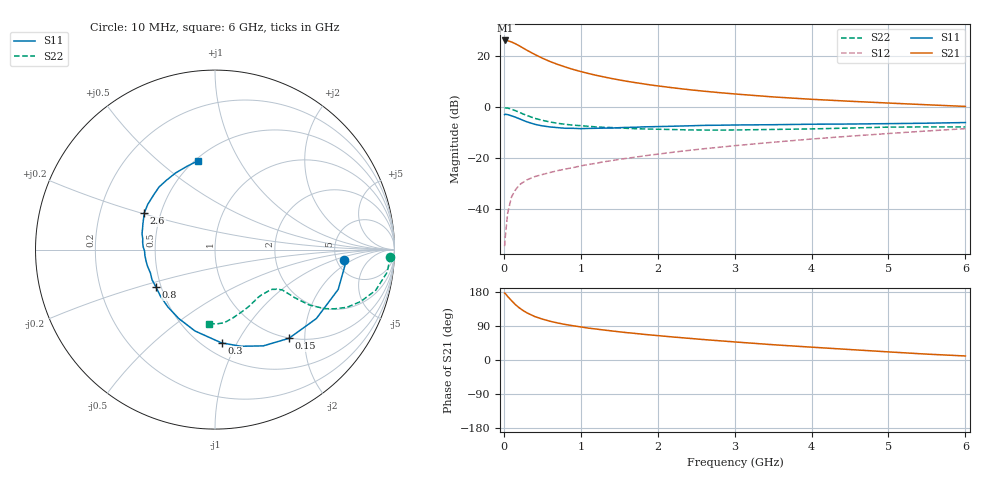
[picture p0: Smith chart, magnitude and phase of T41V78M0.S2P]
! Infineon Technologies  Discrete & RF Semiconductors
! BFR182T
! Si NPN RF Bipolar Junction Transistor in SC75
! VCE = 1.75 V  IC = 8 mA
! Common Emitter S-Parameters:  October  1999
# GHz  S  MA  R  50
!  f  S11  S21  S12  S22
! GHz  MAG  ANG  MAG  ANG  MAG  ANG  MAG  ANG
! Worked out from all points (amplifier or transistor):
!   36 points, 10 MHz to 6 GHz, reference 50 ohm
!   highest |S21| = 26.2 dB at 20 MHz (marker M1)
!   |S21| within 3 dB of that: start of sweep to 251.7 MHz
!   unconditionally stable (mu >= 1): 1.06 GHz to 3.891 GHz
!   at 250 MHz: K = 0.40, MSG = 26.3 dB, |S12| = -29.4 dB
!   at 1.4 GHz: K = 1.08, MAG = 14.4 dB, |S12| = -20.9 dB
!   at 6 GHz: K = 0.85, MSG = 4.4 dB, |S12| = -8.3 dB
!   lowest NFmin = 1.40 dB at 450 MHz
!   S11 on the Smith chart (normalised r, x): 10 MHz: 5.81, -1.47; 150 MHz: 0.99, -1.67; 300 MHz: 0.61, -0.87; 800 MHz: 0.47, -0.23; 2.6 GHz: 0.40, +0.21; 6 GHz: 0.52, +0.69
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0.01  0.722 -4.8  20.52 176.7  0.0019 84.7  0.9757 -2.3
0.02  0.7313 -6.0  20.52 175.3  0.003 95.7  0.9763 -3.0
0.05  0.7214 -17.9  20.27 167.7  0.0085 84.4  0.9674 -7.5
0.1  0.6832 -34.2  19.14 156.6  0.0176 75.7  0.9237 -14.2
0.15  0.6434 -50.2  17.7 146.2  0.0239 69.1  0.8622 -19.6
0.2  0.6 -63.4  16.15 137.7  0.0302 65.3  0.8029 -23.6
0.25  0.5575 -75.0  14.58 130.6  0.0339 60.7  0.7424 -26.4
0.3  0.5211 -86.0  13.21 124.5  0.0379 58.6  0.694 -28.3
0.4  0.467 -103.8  10.95 114.9  0.0439 56.3  0.6111 -30.4
0.5  0.4337 -117.8  9.239 108.0  0.0482 55.8  0.5575 -30.8
0.6  0.4136 -129.3  7.936 102.3  0.0528 55.5  0.5178 -31.1
0.7  0.4005 -139.0  6.96 97.7  0.0575 56.7  0.4874 -31.0
0.8  0.3895 -147.5  6.19 93.7  0.0619 57.1  0.4657 -31.0
1.1  0.3872 -166.1  4.62 84.1  0.0759 60.1  0.4257 -31.6
1.3  0.3919 -175.3  3.96 79.1  0.0859 61.4  0.4071 -32.6
1.6  0.4054 174.1  3.249 72.2  0.1005 62.8  0.3887 -34.7
2.2  0.4272 160.0  2.418 60.7  0.132 64.3  0.3678 -41.5
2.6  0.444 152.6  2.078 53.9  0.1545 64.6  0.3595 -46.7
3.5  0.4575 138.5  1.604 40.3  0.2073 62.6  0.3691 -59.7
4.5  0.4716 125.1  1.319 27.6  0.2728 58.5  0.3933 -75.2
5.5  0.4898 108.5  1.125 15.5  0.3447 53.0  0.4143 -88.7
6  0.5042 100.6  1.045 10.6  0.3826 49.2  0.4135 -94.4
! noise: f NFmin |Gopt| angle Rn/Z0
0.45  1.4  0.26  41  0.29
0.9  1.5  0.25  83  0.23
1.8  2  0.21  162  0.2
